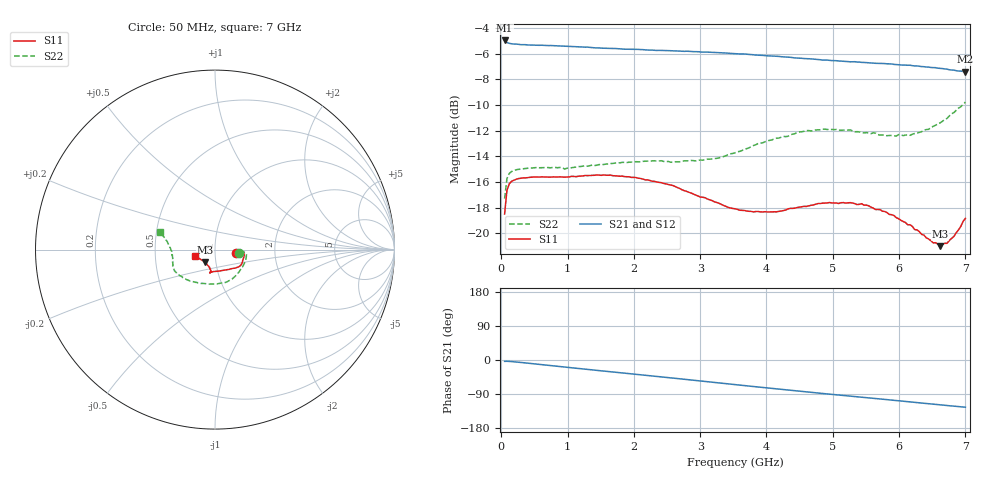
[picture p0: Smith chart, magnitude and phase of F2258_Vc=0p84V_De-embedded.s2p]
! Integrated Device Technology
! Corporate Headquarters
! 6024 Silver Creek Valley Road
! San Jose, CA 95138  USA
! Phone:  1-408-284-8200
! Toll Free:  1-800-223-1366
! Webpage:  http://www.idt.com/
! Timing and RF Division
! 515 Groton Road, Suite 102
! Westford, MA 01886-6024
! Device:  F2258
! Description: Voltage Variable RF Attenuator
! Frequency:  50.0 -  6000.00 MHz
! Package:  3x3 mm Thin QFN Plastic Package: 16 pin
! Ports:  2 RF, 2 DC
!  Pin  1  = NC
!  Pin  2  = NC
!  Pin  3  = RF2  = Port 2
!  Pin  4  = GND
!  Pin  5  = Vdd
!  Pin  6  = NC
!  Pin  7  = VCTRL
!  Pin  8  = NC
!  Pin  9  = GND
!  Pin 10  = RF1  = Port 1
!  Pin 11  = NC
!  Pin 12  = NC
!  Pin 13  = NC
!  Pin 14  = NC
!  Pin 15  = NC
!  Pin 16  = NC
! Vcntrl:  0.840 Volts
! Vdd:  +3.300 Volts
! Current:  1.139 mA
! Data:  The device was measured on a the F2258 evaluation board which has
!  individual transmission lines to the RF pins.  Data was collected
!  using a calibrated network analyzer.  The evaluation board was
!  de-embedded using a TRL calibration technique.
!  The reference plane is the edge of the package pin.
! Misc:  SN 10
!  Action Tracker AT0285
! Date Measured:  2014-12-10
! Date:  2016-01-13  MJV
! Note:
!  Integrated Device Technology supplies this data as a sample of measured
!  data at the package pin for this product.  Your particular data for this
!  product may vary.
!  Data was taken at 25 degrees C.
!  Integrated Device Technology reserves the right to change this data at anytime.
!Freq_(GHz)  S11M_(dB)  S11P_(deg)  S21M_(dB)  S21P_(deg)  S12M_(dB)  S12P_(deg)  S22M_(dB)  S22P_(deg)
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# GHz S dB R 50
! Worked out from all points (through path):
!   201 points, 50 MHz to 7 GHz, reference 50 ohm
!   highest |S21| = -4.97 dB at 50 MHz (marker M1); lowest = -7.4 dB at 7 GHz (marker M2)
!   group delay of S21, straight-line fit = 49.2 ps
!   lowest |S11| = -21.0 dB at 6.618 GHz (marker M3), VSWR 1.20, Z = 44.3 - j6.19 ohm
!   |S11| at or under -10 dB: start of sweep to end of sweep
!   |S22| runs from -17.3 to -9.8 dB; largest |S21 - S12| = 0.0025
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0.05  -18.49 -8.2  -4.97 -3.5  -4.98 -3.6  -17.29 -7.2
0.08475  -16.66 -4.9  -5.13 -3.4  -5.14 -3.4  -15.74 -5.3
0.1195  -16.15 -4.2  -5.19 -3.6  -5.21 -3.7  -15.34 -5.8
0.15425  -15.94 -4.4  -5.23 -4.1  -5.24 -4.1  -15.18 -6.9
0.5365  -15.60 -11.5  -5.35 -10.9  -5.37 -10.9  -14.87 -19.0
0.9535  -15.62 -20.8  -5.41 -18.5  -5.44 -18.5  -14.98 -33.6
1.2315  -15.52 -25.1  -5.48 -23.6  -5.50 -23.6  -14.76 -42.5
1.6485  -15.46 -30.7  -5.59 -31.0  -5.60 -31.0  -14.56 -54.4
2.37825  -16.02 -38.7  -5.74 -43.9  -5.74 -43.9  -14.36 -74.2
3.0385  -17.18 -51.5  -5.88 -55.9  -5.87 -55.9  -14.30 -96.4
3.525  -18.08 -67.8  -6.00 -64.9  -6.00 -64.9  -13.72 -115.7
3.803  -18.32 -79.6  -6.08 -70.0  -6.09 -70.0  -13.16 -126.2
4.1505  -18.32 -91.3  -6.20 -76.2  -6.21 -76.2  -12.58 -136.7
4.7065  -17.78 -101.7  -6.42 -86.0  -6.41 -86.0  -12.00 -149.7
5.2625  -17.60 -102.9  -6.64 -95.3  -6.61 -95.3  -11.94 -158.9
5.43625  -17.68 -101.6  -6.68 -98.2  -6.65 -98.2  -12.15 -161.7
5.85325  -18.52 -101.5  -6.79 -105.2  -6.78 -105.2  -12.37 -170.2
6.166  -19.32 -105.1  -6.90 -110.5  -6.90 -110.5  -12.36 -177.4
6.61775  -20.99 -129.0  -7.14 -118.2  -7.11 -118.3  -11.39 170.5
6.722  -20.77 -137.9  -7.20 -120.0  -7.19 -120.1  -11.05 167.7
6.82625  -20.23 -146.9  -7.28 -121.7  -7.26 -121.8  -10.59 165.8
7  -18.83 -162.0  -7.40 -124.6  -7.40 -124.6  -9.77 162.1
